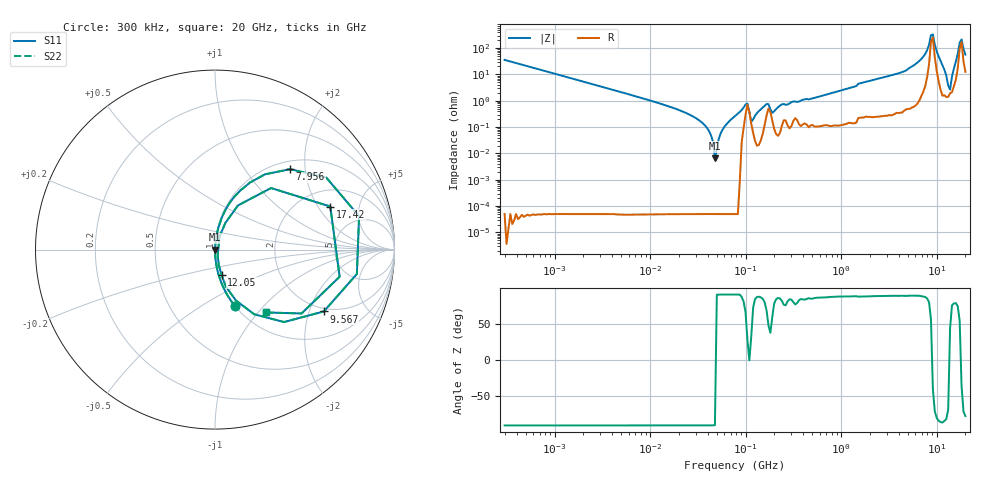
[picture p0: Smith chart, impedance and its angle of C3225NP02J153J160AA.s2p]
! S-parameter Generated by TDK Corporation
! Copyright(C) 2015 TDK Corporation.
! All Rights Reserved.
! TDK P/N: C3225NP02J153J160AA (Multilayer Ceramic Chip Capacitors)
! Property: C=15nF
! Size(LxWxT): 3.2x2.5x1.6mm, 0.126x0.098x0.063inches
! Model Type: s2p (Touchstone File Format Version 1.0)
! Frequency: DC=Yes Start=0.3MHz Stop=20000MHz 243points Log-sweep
! Note:
! Model Generated on Jun. 23, 2015
! Hash(MD5):
! Port Assignments:
!  1 ---| |--- 2
! Applicable Conditions:
!  Temperature = 25 degC
!  DC Bias Voltage = 0 V
!  Small Signal Operation
! Terms and conditions regarding TDK Simulation Models
! (1)This simulation model is being provided solely for informational purposes. Please refer to the specifications of the products in terms of detailed characteristics of such products.
! (2)In no event shall TDK Corporation of any of its subsidiaries be liable for any loss or damage arising, directly or indirectly,
!  From any information contained in this simulation model, including, but not limited to loss or damages arising from any inaccuracies, omissions or errors in connection with such information.
! (3)Any and all copyrights on this simulation model are owned by TDK Corporation.
!  Duplication or redistribution of this simulation model without prior written permission from TDK Corporation is prohibited.
! (4)This simulation model is subject to any modification or change without any prior notice.
! (5)Neither TDK Corporation nor any of its subsidiaries shall make any warranty, express or implied,
!  Including but not limited to the correctness, implied warranties of merchantability and fitness for a particular purpose with respect to this simulation models.
! (6)The use of this simulation model shall be deemed to have consented to the terms and conditions hereof.
# MHz S MA R 50
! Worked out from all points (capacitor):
!   242 points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, 300 kHz to 20 GHz, reference 50 ohm
!   read as one part in series: C = 14.9 nF near 314.2 kHz
!   lowest |Z| = 6.43 mohm at 47.74 MHz (marker M1)
!   series resonance near 48.44 MHz, so ESL is about 730 pH
!   S11 on the Smith chart (normalised r, x): 300 kHz: 1.00, -0.71; 7.956 GHz: 1.16, +1.66; 9.567 GHz: 1.88, -2.52; 12.05 GHz: 1.03, -0.30; 17.42 GHz: 2.85, +2.59; 20 GHz: 1.25, -1.10
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0.3  0.3355 -70.4  0.942 19.6  0.942 19.6  0.3355 -70.4
1.985118  0.05372 -86.9  0.9986 3.1  0.9986 3.1  0.05372 -86.9
12.54397  0.00797 -90.6  0.9998 0.5  0.9998 0.5  0.00797 -90.6
34.57736  0.001545 -96.0  0.9998 0.1  0.9998 0.1  0.001545 -96.0
47.74252  0.0001704 -158.0  0.9998 0.0  0.9998 0.0  0.0001704 -158.0
57.40771  0.0008187 100.3  0.9999 -0.0  0.9999 -0.0  0.0008187 100.3
79.26541  0.002818 92.0  0.9999 -0.2  0.9999 -0.2  0.002818 92.0
104.5156  0.007769 27.8  0.9931 -0.2  0.9931 -0.2  0.007769 27.8
114.6076  0.001594 32.3  0.9987 -0.0  0.9987 -0.0  0.001594 32.3
165.7079  0.007503 68.0  0.9972 -0.4  0.9972 -0.4  0.007503 68.0
190.2795  0.003473 59.0  0.9982 -0.2  0.9982 -0.2  0.003473 59.0
500.8786  0.01215 83.6  0.9987 -0.7  0.9987 -0.7  0.01215 83.6
3165.055  0.08699 83.1  0.9934 -5.0  0.9934 -5.0  0.08699 83.1
6318.653  0.2727 72.6  0.9546 -15.8  0.9546 -15.8  0.2727 72.6
7956.199  0.6127 47.0  0.7337 -37.6  0.7337 -37.6  0.6127 47.0
9135.962  0.8021 -9.7  0.2437 30.7  0.2437 30.7  0.8021 -9.7
9566.884  0.6974 -29.6  0.5205 41.0  0.5205 41.0  0.6974 -29.6
12046.24  0.1463 -75.4  0.9735 8.4  0.9735 8.4  0.1463 -75.4
13832.49  0.02546 41.1  0.981 -1.1  0.981 -1.1  0.02546 41.1
15883.6  0.2775 62.5  0.9051 -15.8  0.9051 -15.8  0.2775 62.5
17417.32  0.6857 20.5  0.4297 -33.7  0.4297 -33.7  0.6857 20.5
20000  0.45 -51.1  0.7983 26.0  0.7983 26.0  0.45 -51.1
